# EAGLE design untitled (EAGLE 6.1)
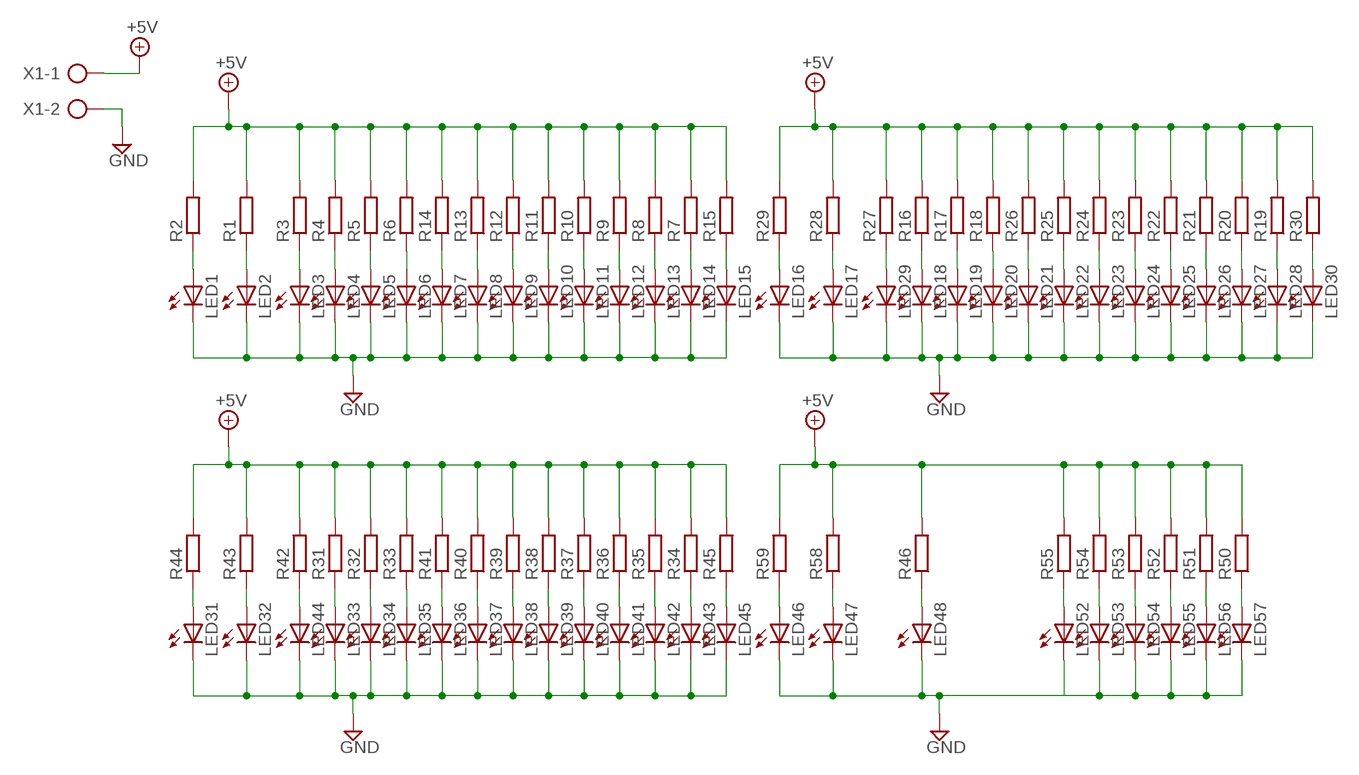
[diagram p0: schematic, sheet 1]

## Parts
LED1  LED5MM  [LED5MM]
LED2  LED5MM  [LED5MM]
LED3  LED5MM  [LED5MM]
LED4  LED5MM  [LED5MM]
LED5  LED5MM  [LED5MM]
LED6  LED5MM  [LED5MM]
LED7  LED5MM  [LED5MM]
LED8  LED5MM  [LED5MM]
LED9  LED5MM  [LED5MM]
LED10  LED5MM  [LED5MM]
LED11  LED5MM  [LED5MM]
LED12  LED5MM  [LED5MM]
LED13  LED5MM  [LED5MM]
LED14  LED5MM  [LED5MM]
LED15  LED5MM  [LED5MM]
LED16  LED5MM  [LED5MM]
LED17  LED5MM  [LED5MM]
LED18  LED5MM  [LED5MM]
LED19  LED5MM  [LED5MM]
LED20  LED5MM  [LED5MM]
LED21  LED5MM  [LED5MM]
LED22  LED5MM  [LED5MM]
LED23  LED5MM  [LED5MM]
LED24  LED5MM  [LED5MM]
LED25  LED5MM  [LED5MM]
LED26  LED5MM  [LED5MM]
LED27  LED5MM  [LED5MM]
LED28  LED5MM  [LED5MM]
LED29  LED5MM  [LED5MM]
LED30  LED5MM  [LED5MM]
LED31  LED5MM  [LED5MM]
LED32  LED5MM  [LED5MM]
LED33  LED5MM  [LED5MM]
LED34  LED5MM  [LED5MM]
LED35  LED5MM  [LED5MM]
LED36  LED5MM  [LED5MM]
LED37  LED5MM  [LED5MM]
LED38  LED5MM  [LED5MM]
LED39  LED5MM  [LED5MM]
LED40  LED5MM  [LED5MM]
LED41  LED5MM  [LED5MM]
LED42  LED5MM  [LED5MM]
LED43  LED5MM  [LED5MM]
LED44  LED5MM  [LED5MM]
LED45  LED5MM  [LED5MM]
LED46  LED5MM  [LED5MM]
LED47  LED5MM  [LED5MM]
LED48  LED5MM  [LED5MM]
LED52  LED5MM  [LED5MM]
LED53  LED5MM  [LED5MM]
LED54  LED5MM  [LED5MM]
LED55  LED5MM  [LED5MM]
LED56  LED5MM  [LED5MM]
LED57  LED5MM  [LED5MM]
R1  R-EU_0207/15  [0207/15]
R2  R-EU_0207/15  [0207/15]
R3  R-EU_0207/15  [0207/15]
R4  R-EU_0207/15  [0207/15]
R5  R-EU_0207/15  [0207/15]
R6  R-EU_0207/15  [0207/15]
R7  R-EU_0207/15  [0207/15]
R8  R-EU_0207/15  [0207/15]
R9  R-EU_0207/15  [0207/15]
R10  R-EU_0207/15  [0207/15]
R11  R-EU_0207/15  [0207/15]
R12  R-EU_0207/15  [0207/15]
R13  R-EU_0207/15  [0207/15]
R14  R-EU_0207/15  [0207/15]
R15  R-EU_0207/15  [0207/15]
R16  R-EU_0207/15  [0207/15]
R17  R-EU_0207/15  [0207/15]
R18  R-EU_0207/15  [0207/15]
R19  R-EU_0207/15  [0207/15]
R20  R-EU_0207/15  [0207/15]
R21  R-EU_0207/15  [0207/15]
R22  R-EU_0207/15  [0207/15]
R23  R-EU_0207/15  [0207/15]
R24  R-EU_0207/15  [0207/15]
R25  R-EU_0207/15  [0207/15]
R26  R-EU_0207/15  [0207/15]
R27  R-EU_0207/15  [0207/15]
R28  R-EU_0207/15  [0207/15]
R29  R-EU_0207/15  [0207/15]
R30  R-EU_0207/15  [0207/15]
R31  R-EU_0207/15  [0207/15]
R32  R-EU_0207/15  [0207/15]
R33  R-EU_0207/15  [0207/15]
R34  R-EU_0207/15  [0207/15]
R35  R-EU_0207/15  [0207/15]
R36  R-EU_0207/15  [0207/15]
R37  R-EU_0207/15  [0207/15]
R38  R-EU_0207/15  [0207/15]
R39  R-EU_0207/15  [0207/15]
R40  R-EU_0207/15  [0207/15]
R41  R-EU_0207/15  [0207/15]
R42  R-EU_0207/15  [0207/15]
R43  R-EU_0207/15  [0207/15]
R44  R-EU_0207/15  [0207/15]
R45  R-EU_0207/15  [0207/15]
R46  R-EU_0207/15  [0207/15]
R50  R-EU_0207/15  [0207/15]
R51  R-EU_0207/15  [0207/15]
R52  R-EU_0207/15  [0207/15]
R53  R-EU_0207/15  [0207/15]
R54  R-EU_0207/15  [0207/15]
R55  R-EU_0207/15  [0207/15]
R58  R-EU_0207/15  [0207/15]
R59  R-EU_0207/15  [0207/15]
X1  AK300/2  [AK300/2]

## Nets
+5V: R1.2 R2.2 R3.2 R4.2 R5.2 R6.2 R7.2 R8.2 R9.2 R10.2 R11.2 R12.2 R13.2 R14.2 R15.2 R16.2 R17.2 R18.2 R19.2 R20.2 R21.2 R22.2 R23.2 R24.2 R25.2 R26.2 R27.2 R28.2 R29.2 R30.2 R31.2 R32.2 R33.2 R34.2 R35.2 R36.2 R37.2 R38.2 R39.2 R40.2 R41.2 R42.2 R43.2 R44.2 R45.2 R46.2 R50.2 R51.2 R52.2 R53.2 R54.2 R55.2 R58.2 R59.2 X1.1
GND: LED1.K(C) LED2.K(C) LED3.K(C) LED4.K(C) LED5.K(C) LED6.K(C) LED7.K(C) LED8.K(C) LED9.K(C) LED10.K(C) LED11.K(C) LED12.K(C) LED13.K(C) LED14.K(C) LED15.K(C) LED16.K(C) LED17.K(C) LED18.K(C) LED19.K(C) LED20.K(C) LED21.K(C) LED22.K(C) LED23.K(C) LED24.K(C) LED25.K(C) LED26.K(C) LED27.K(C) LED28.K(C) LED29.K(C) LED30.K(C) LED31.K(C) LED32.K(C) LED33.K(C) LED34.K(C) LED35.K(C) LED36.K(C) LED37.K(C) LED38.K(C) LED39.K(C) LED40.K(C) LED41.K(C) LED42.K(C) LED43.K(C) LED44.K(C) LED45.K(C) LED46.K(C) LED47.K(C) LED48.K(C) LED52.K(C) LED53.K(C) LED54.K(C) LED55.K(C) LED56.K(C) LED57.K(C) X1.2
N$1: LED15.A R15.1
N$2: LED1.A R2.1
N$3: LED2.A R1.1
N$4: LED3.A R3.1
N$5: LED4.A R4.1
N$6: LED5.A R5.1
N$7: LED6.A R6.1
N$8: LED7.A R14.1
N$9: LED8.A R13.1
N$10: LED9.A R12.1
N$11: LED10.A R11.1
N$12: LED11.A R10.1
N$13: LED12.A R9.1
N$14: LED13.A R8.1
N$15: LED14.A R7.1
N$16: LED16.A R29.1
N$17: LED17.A R28.1
N$18: LED29.A R27.1
N$19: LED18.A R16.1
N$20: LED19.A R17.1
N$21: LED20.A R18.1
N$22: LED21.A R26.1
N$23: LED22.A R25.1
N$24: LED23.A R24.1
N$25: LED24.A R23.1
N$26: LED25.A R22.1
N$27: LED26.A R21.1
N$28: LED27.A R20.1
N$29: LED28.A R19.1
N$30: LED30.A R30.1
N$31: LED31.A R44.1
N$32: LED32.A R43.1
N$33: LED44.A R42.1
N$34: LED33.A R31.1
N$35: LED34.A R32.1
N$36: LED35.A R33.1
N$37: LED36.A R41.1
N$38: LED37.A R40.1
N$39: LED38.A R39.1
N$40: LED39.A R38.1
N$41: LED40.A R37.1
N$42: LED41.A R36.1
N$43: LED42.A R35.1
N$44: LED43.A R34.1
N$45: LED45.A R45.1
N$46: LED46.A R59.1
N$47: LED47.A R58.1
N$49: LED48.A R46.1
N$53: LED52.A R55.1
N$54: LED53.A R54.1
N$55: LED54.A R53.1
N$56: LED55.A R52.1
N$57: LED56.A R51.1
N$58: LED57.A R50.1

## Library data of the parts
LED1-LED48 LED52-LED57 = led:LED: LED
R1-R46 R50-R55 R58 R59 = rcl:R-EU_: RESISTOR, European symbol
X1 = con-ptr500:AK300/2: CONNECTOR; OC_FARNELL: unknown; OC_NEWARK: unknown

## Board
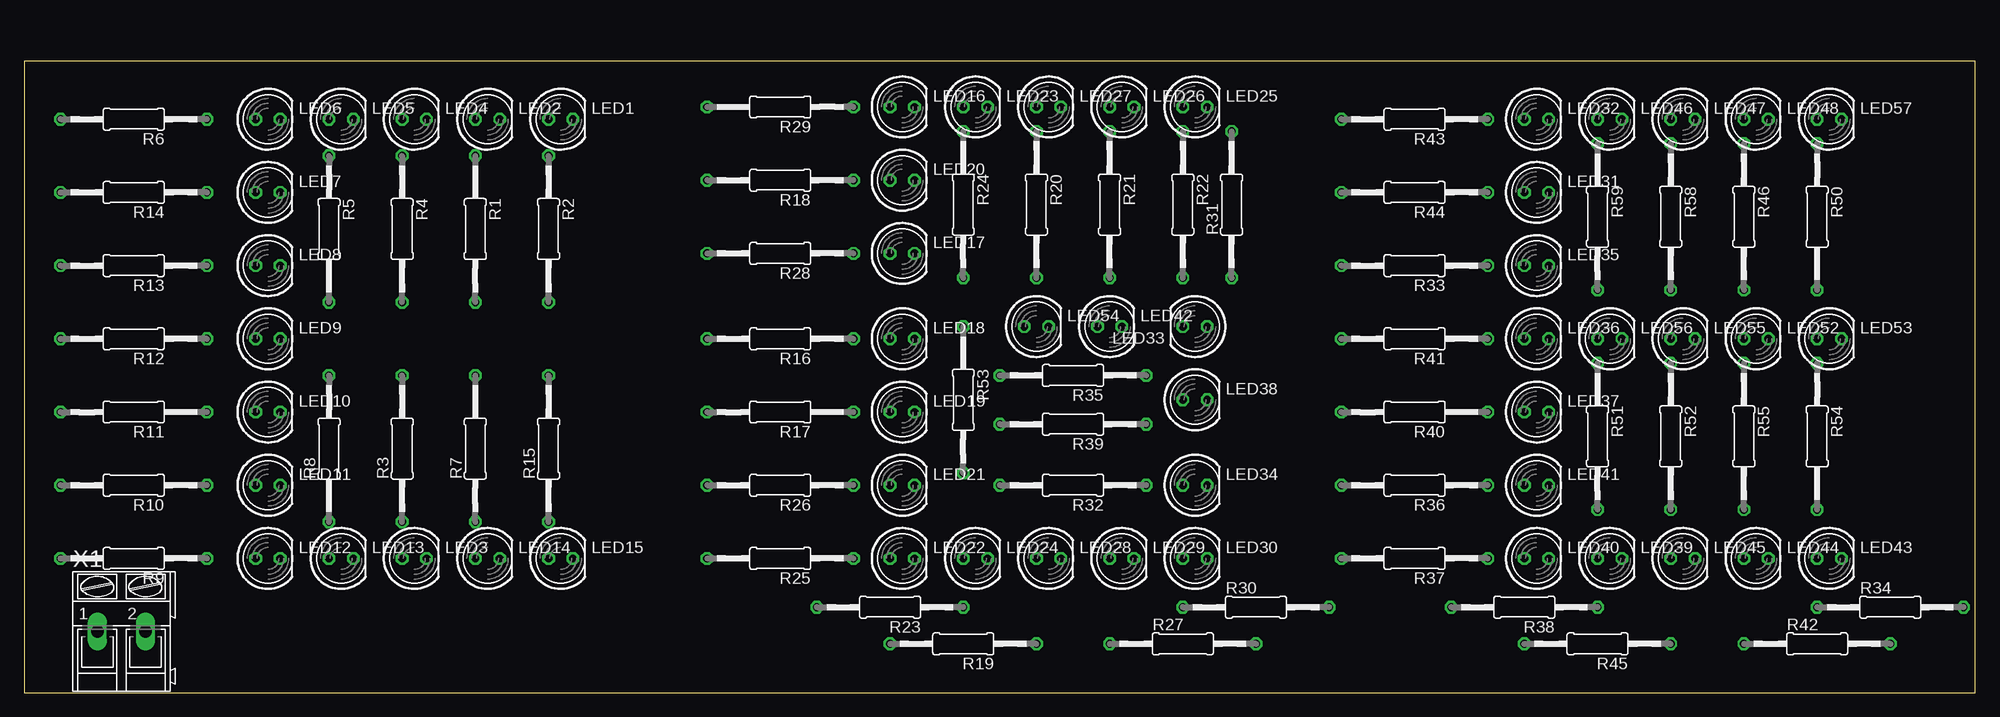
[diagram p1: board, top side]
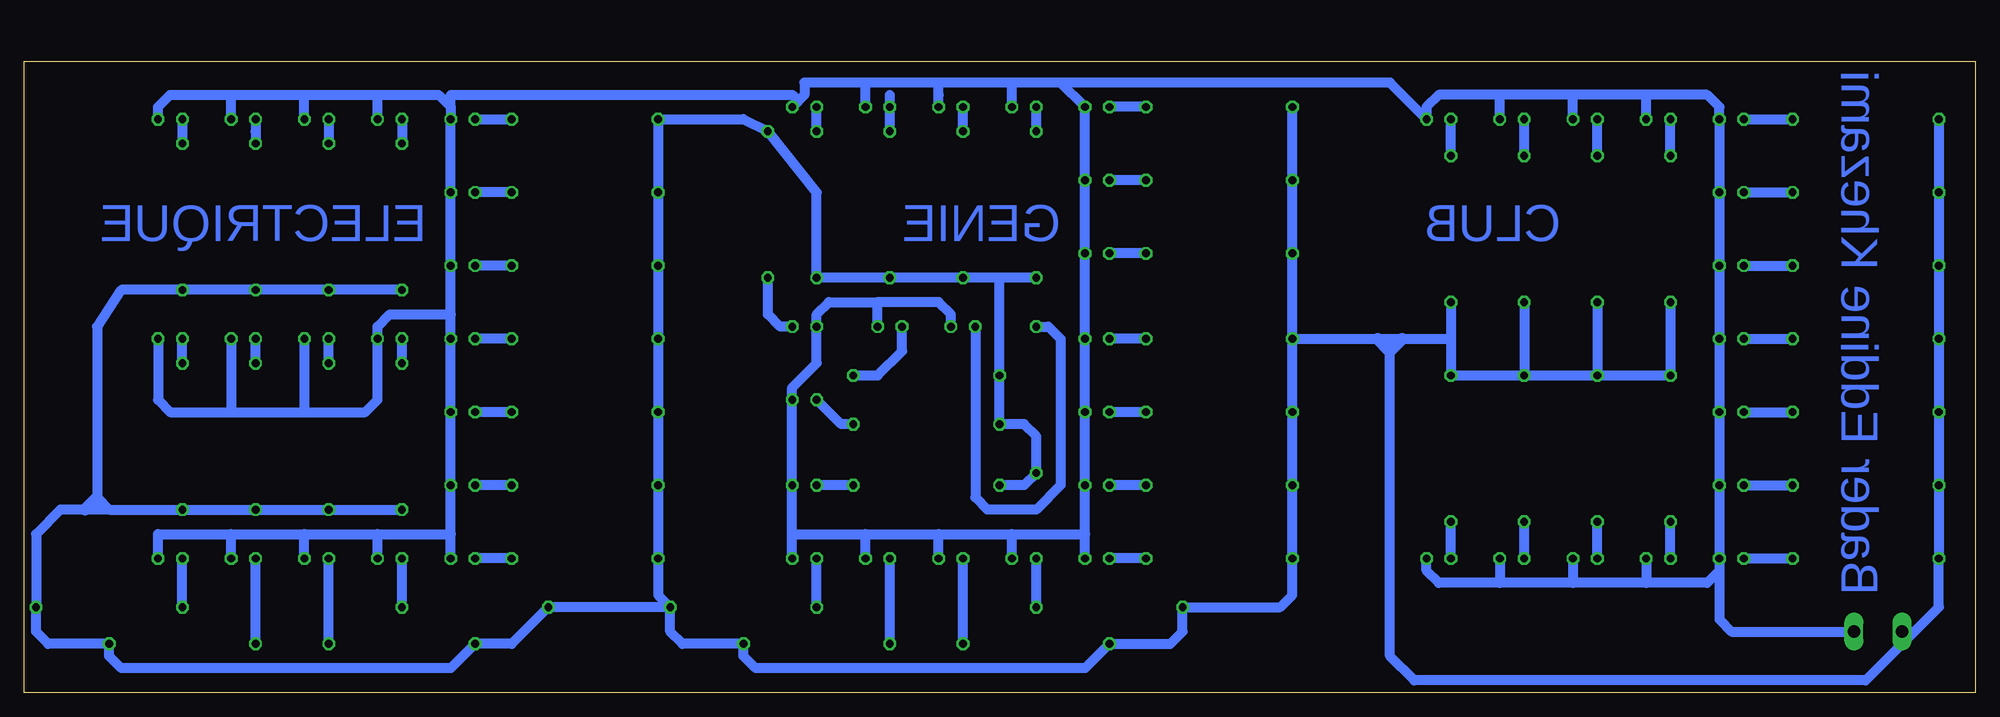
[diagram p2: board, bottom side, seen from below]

Size 203.18 x 65.71 mm. Coordinates in mm from the lower left corner, seen from the top.
Outline: 0,0 203.18,0 203.18,65.71 0,65.71 0,0
Copper layers (1*16): Top 0.035mm / dielectric 1.5mm / Bottom 0.035mm
Design rules: minimum track width 10mil, minimum drill 24mil, track to track 8mil, track to pad 8mil, pad to pad 8mil, via to via 8mil, smd to smd 8mil, copper to edge 40mil, drill to drill 8mil, minimum pad ring 10mil, minimum via ring 8mil, stop-mask expansion 4mil, vias tented up to drill 0mil, thermal gap 10mil

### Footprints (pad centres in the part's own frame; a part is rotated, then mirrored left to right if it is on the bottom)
LED5MM = drill 0.813 octagon: A -1.27,0; K 1.27,0
0207/15 = drill 0.813 octagon: 1 -7.62,0; 2 7.62,0
AK300/2 = drill 1.321 long: 1 -2.515,0; 2 2.489,0

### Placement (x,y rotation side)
LED1  55.88,59.69 0 top
LED2  48.26,59.69 0 top
LED3  40.64,13.97 0 top
LED4  40.64,59.69 0 top
LED5  33.02,59.69 0 top
LED6  25.4,59.69 0 top
LED7  25.4,52.07 0 top
LED8  25.4,44.45 0 top
LED9  25.4,36.83 0 top
LED10  25.4,29.21 0 top
LED11  25.4,21.59 0 top
LED12  25.4,13.97 0 top
LED13  33.02,13.97 0 top
LED14  48.26,13.97 0 top
LED15  55.88,13.97 0 top
LED16  91.44,60.96 0 top
LED17  91.44,45.72 0 top
LED18  91.44,36.83 0 top
LED19  91.44,29.21 0 top
LED20  91.44,53.34 0 top
LED21  91.44,21.59 0 top
LED22  91.44,13.97 0 top
LED23  99.06,60.96 0 top
LED24  99.06,13.97 0 top
LED25  121.92,60.96 0 top
LED26  114.3,60.96 0 top
LED27  106.68,60.96 0 top
LED28  106.68,13.97 0 top
LED29  114.3,13.97 0 top
LED30  121.92,13.97 0 top
LED31  157.48,52.07 0 top
LED32  157.48,59.69 0 top
LED33  121.92,38.1 180 top
LED34  121.92,21.59 0 top
LED35  157.48,44.45 0 top
LED36  157.48,36.83 0 top
LED37  157.48,29.21 0 top
LED38  121.92,30.48 0 top
LED39  165.1,13.97 0 top
LED40  157.48,13.97 0 top
LED41  157.48,21.59 0 top
LED42  113.03,38.1 0 top
LED43  187.96,13.97 0 top
LED44  180.34,13.97 0 top
LED45  172.72,13.97 0 top
LED46  165.1,59.69 0 top
LED47  172.72,59.69 0 top
LED48  180.34,59.69 0 top
LED52  180.34,36.83 0 top
LED53  187.96,36.83 0 top
LED54  105.41,38.1 0 top
LED55  172.72,36.83 0 top
LED56  165.1,36.83 0 top
LED57  187.96,59.69 0 top
R1  46.99,48.26 270 top
R2  54.61,48.26 270 top
R3  39.37,25.4 90 top
R4  39.37,48.26 270 top
R5  31.75,48.26 270 top
R6  11.43,59.69 180 top
R7  46.99,25.4 90 top
R8  31.75,25.4 90 top
R9  11.43,13.97 180 top
R10  11.43,21.59 180 top
R11  11.43,29.21 180 top
R12  11.43,36.83 180 top
R13  11.43,44.45 180 top
R14  11.43,52.07 180 top
R15  54.61,25.4 90 top
R16  78.74,36.83 180 top
R17  78.74,29.21 180 top
R18  78.74,53.34 180 top
R19  97.79,5.08 180 top
R20  105.41,50.8 270 top
R21  113.03,50.8 270 top
R22  120.65,50.8 270 top
R23  90.17,8.89 180 top
R24  97.79,50.8 270 top
R25  78.74,13.97 180 top
R26  78.74,21.59 180 top
R27  120.65,5.08 0 top
R28  78.74,45.72 180 top
R29  78.74,60.96 180 top
R30  128.27,8.89 0 top
R31  125.73,50.8 90 top
R32  109.22,21.59 180 top
R33  144.78,44.45 180 top
R34  194.31,8.89 0 top
R35  109.22,33.02 180 top
R36  144.78,21.59 180 top
R37  144.78,13.97 180 top
R38  156.21,8.89 180 top
R39  109.22,27.94 180 top
R40  144.78,29.21 180 top
R41  144.78,36.83 180 top
R42  186.69,5.08 0 top
R43  144.78,59.69 180 top
R44  144.78,52.07 180 top
R45  163.83,5.08 180 top
R46  179.07,49.53 270 top
R50  186.69,49.53 270 top
R51  163.83,26.67 270 top
R52  171.45,26.67 270 top
R53  97.79,30.48 270 top
R54  186.69,26.67 270 top
R55  179.07,26.67 270 top
R58  171.45,49.53 270 top
R59  163.83,49.53 270 top
X1  10.16,6.35 0 top

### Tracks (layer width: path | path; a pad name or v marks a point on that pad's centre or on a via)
+5V
  Bottom 1.016: R6.2 R14.2 R13.2 R12.2 | R12.2 R11.2 R10.2 R9.2 | R5.2 R8.2 R3.2 | R4.2 R3.2 | R1.2 R7.2 | R2.2 54.61,36.83 | 54.61,36.83 R15.2 R7.2 | R7.2 R3.2 | R16.2 R17.2 R26.2 R25.2 71.12,10.16 72.39,8.89 R23.2 82.55,6.35 83.82,5.08 R19.2 92.71,2.54 127,2.54 128.27,3.81 R27.2 134.62,5.08 135.89,6.35 R30.2 | R16.2 R28.2 R18.2 R29.2 | R16.2 62.23,36.83 60.96,36.83 | 60.96,36.83 59.69,36.83 54.61,36.83 | R24.2 101.6,43.18 | 101.6,43.18 R20.2 R21.2 R22.2 120.65,52.07 R31.2 128.27,59.69 R43.2 R44.2 R33.2 R41.2 R40.2 R36.2 R37.2 137.16,10.16 R30.2 | R32.2 99.06,21.59 R53.2 97.79,26.67 99.06,27.94 R39.2 R35.2 101.6,43.18 | R59.2 R58.2 R46.2 R50.2 193.04,41.91 195.58,38.1 195.58,20.32 194.31,19.05 | 194.31,19.05 R54.2 R55.2 R52.2 R51.2 | 194.31,19.05 196.85,19.05 199.39,19.05 201.93,16.51 R34.2 201.93,6.35 200.66,5.08 R42.2 194.31,3.81 193.04,2.54 158.75,2.54 R45.2 152.4,5.08 R38.2 R30.2 | X1.1 6.35,6.35 | 6.35,6.35 3.81,8.89 R9.2 | R12.2 R9.2 | 6.35,6.35 11.43,1.27 58.42,1.27 60.96,3.81 60.96,35.56 60.96,36.83
  Bottom 1.27: 59.69,36.83 60.96,35.56 62.23,36.83 | 195.58,20.32 196.85,19.05
GND
  Bottom 1.016: 34.29,62.23 27.94,62.23 26.67,60.96 LED6.K LED7.K LED8.K LED9.K LED10.K LED11.K LED12.K 26.67,12.7 | 34.29,62.23 41.91,62.23 | 41.91,62.23 49.53,62.23 | 49.53,62.23 55.88,62.23 57.15,60.96 LED1.K 60.96,63.5 95.25,63.5 | LED4.K 41.91,62.23 | LED2.K 49.53,62.23 | LED5.K 34.29,62.23 | 26.67,12.7 27.94,11.43 34.29,11.43 | 34.29,11.43 41.91,11.43 | 41.91,11.43 49.53,11.43 | 49.53,11.43 55.88,11.43 57.15,12.7 LED15.K | LED14.K 49.53,11.43 | LED3.K 41.91,11.43 | LED13.K 34.29,11.43 | LED22.K 92.71,16.51 | 92.71,16.51 LED21.K LED19.K LED18.K LED17.K LED20.K LED16.K 95.25,63.5 | 95.25,63.5 100.33,63.5 | 100.33,63.5 107.95,63.5 | 107.95,63.5 115.57,63.5 | 115.57,63.5 121.92,63.5 121.92,62.23 122.55,61.6 | 122.55,61.6 LED25.K | LED23.K 100.33,63.5 | 107.95,62.23 LED27.K 107.95,63.5 | LED26.K 115.57,63.5 | 123.19,16.51 LED34.K LED38.K 123.19,31.75 120.65,34.29 LED33.K 120.65,39.37 119.38,40.64 114.3,40.64 | LED40.K 158.75,16.51 | 158.75,16.51 LED41.K LED37.K LED36.K 158.75,39.37 | 158.75,39.37 LED35.K LED31.K LED32.K 158.75,60.96 | LED57.K 189.23,60.96 187.96,62.23 181.61,62.23 | 181.61,62.23 173.99,62.23 | 173.99,62.23 166.37,62.23 | 166.37,62.23 160.02,62.23 158.75,60.96 | LED46.K 166.37,62.23 | LED47.K 173.99,62.23 | LED48.K 181.61,62.23 | LED53.K 189.23,30.48 187.96,29.21 181.61,29.21 | 181.61,29.21 173.99,29.21 | 173.99,29.21 167.64,29.21 166.37,30.48 LED56.K 166.37,38.1 165.1,39.37 158.75,39.37 | LED55.K 173.99,29.21 | LED52.K 181.61,29.21 | 158.75,60.96 158.75,62.23 123.19,62.23 122.55,61.6 | LED43.K 189.23,16.51 181.61,16.51 | 181.61,16.51 173.99,16.51 | 173.99,16.51 166.37,16.51 | 166.37,16.51 158.75,16.51 | LED44.K 181.61,16.51
  Bottom 1.016: LED45.K 173.99,16.51 | LED39.K 166.37,16.51 | 26.67,12.7 26.67,7.62 25.4,6.35 X1.2 | LED54.K 106.68,39.37 107.95,40.64 114.3,40.64 | LED42.K 114.3,40.64 | LED30.K 123.19,16.51 | 123.19,16.51 115.57,16.51 | 115.57,16.51 107.95,16.51 | 107.95,16.51 100.33,16.51 | 100.33,16.51 92.71,16.51 | LED24.K 100.33,16.51 | LED28.K 107.95,16.51 | LED29.K 115.57,16.51
N$1
  Bottom 1.016: LED15.A R15.1
N$2
  Bottom 1.016: R2.1 LED1.A
N$3
  Bottom 1.016: R1.1 LED2.A
N$4
  Bottom 1.016: LED3.A R3.1
N$5
  Bottom 1.016: R4.1 LED4.A
N$6
  Bottom 1.016: R5.1 LED5.A
N$7
  Bottom 1.016: LED6.A R6.1
N$8
  Bottom 1.016: LED7.A R14.1
N$9
  Bottom 1.016: LED8.A R13.1
N$10
  Bottom 1.016: LED9.A R12.1
N$11
  Bottom 1.016: LED10.A R11.1
N$12
  Bottom 1.016: LED11.A R10.1
N$13
  Bottom 1.016: LED12.A R9.1
N$14
  Bottom 1.016: LED13.A R8.1
N$15
  Bottom 1.016: LED14.A R7.1
N$16
  Bottom 1.016: R29.1 LED16.A
N$17
  Bottom 1.016: R28.1 LED17.A
N$18
  Bottom 1.016: R27.1 LED29.A
N$19
  Bottom 1.016: R16.1 LED18.A
N$20
  Bottom 1.016: R17.1 LED19.A
N$21
  Bottom 1.016: R18.1 LED20.A
N$22
  Bottom 1.016: R26.1 LED21.A
N$23
  Bottom 1.016: R25.1 LED22.A
N$24
  Bottom 1.016: R24.1 LED23.A
N$25
  Bottom 1.016: R23.1 LED24.A
N$26
  Bottom 1.016: R22.1 LED25.A
N$27
  Bottom 1.016: 113.03,62.23 LED26.A R21.1
N$28
  Bottom 1.016: R20.1 LED27.A
N$29
  Bottom 1.016: R19.1 LED28.A
N$30
  Bottom 1.016: R30.1 LED30.A
N$31
  Bottom 1.016: R44.1 LED31.A
N$32
  Bottom 1.016: LED32.A R43.1
N$33
  Bottom 1.016: R42.1 LED44.A
N$34
  Bottom 1.016: LED33.A 124.46,38.1 125.73,39.37 R31.1
N$35
  Bottom 1.016: R32.1 LED34.A
N$36
  Bottom 1.016: R33.1 LED35.A
N$37
  Bottom 1.016: R41.1 LED36.A
N$38
  Bottom 1.016: R40.1 LED37.A
N$39
  Bottom 1.016: R39.1 118.11,27.94 LED38.A
N$40
  Bottom 1.016: R38.1 LED39.A
N$41
  Bottom 1.016: R37.1 LED40.A
N$42
  Bottom 1.016: R36.1 LED41.A
N$43
  Bottom 1.016: R35.1 114.3,33.02 111.76,35.56 LED42.A
N$44
  Bottom 1.016: R34.1 LED43.A
N$45
  Bottom 1.016: R45.1 LED45.A
N$46
  Bottom 1.016: LED46.A R59.1
N$47
  Bottom 1.016: LED47.A R58.1
N$49
  Bottom 1.016: LED48.A 179.07,58.42 R46.1
N$53
  Bottom 1.016: R55.1 LED52.A
N$54
  Bottom 1.016: R54.1 LED53.A
N$55
  Bottom 1.016: R53.1 96.52,38.1 95.25,36.83 95.25,21.59 97.79,19.05 102.87,19.05 104.14,20.32 LED54.A
N$56
  Bottom 1.016: R52.1 LED55.A
N$57
  Bottom 1.016: R51.1 LED56.A
N$58
  Bottom 1.016: LED57.A R50.1

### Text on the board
Bottom: CLUB | GENIE | ELECTRIQUE | Bader Eddine Khezami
